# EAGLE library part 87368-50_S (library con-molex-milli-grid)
RECEPTACAL
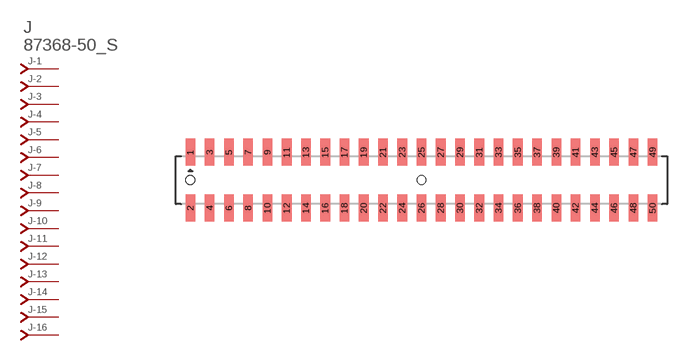
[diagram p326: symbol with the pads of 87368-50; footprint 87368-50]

Designator prefix J; gates -1=J-NV -2=J-N -3=J-N -4=J-N -5=J-N -6=J-N -7=J-N -8=J-N -9=J-N -10=J-N -11=J-N -12=J-N -13=J-N -14=J-N -15=J-N -16=J-N -17=J-N -18=J-N -19=J-N -20=J-N -21=J-N -22=J-N -23=J-N -24=J-N -25=J-N -26=J-N -27=J-N -28=J-N -29=J-N -30=J-N -31=J-N -32=J-N -33=J-N -34=J-N -35=J-N -36=J-N -37=J-N -38=J-N -39=J-N -40=J-N -41=J-N -42=J-N -43=J-N -44=J-N -45=J-N -46=J-N -47=J-N -48=J-N -49=J-N -50=J-N

## 87368-50_S  [87368-50]
1  -1:J  pas
2  -2:J  pas
3  -3:J  pas
4  -4:J  pas
5  -5:J  pas
6  -6:J  pas
7  -7:J  pas
8  -8:J  pas
9  -9:J  pas
10  -10:J  pas
11  -11:J  pas
12  -12:J  pas
13  -13:J  pas
14  -14:J  pas
15  -15:J  pas
16  -16:J  pas
17  -17:J  pas
18  -18:J  pas
19  -19:J  pas
20  -20:J  pas
21  -21:J  pas
22  -22:J  pas
23  -23:J  pas
24  -24:J  pas
25  -25:J  pas
26  -26:J  pas
27  -27:J  pas
28  -28:J  pas
29  -29:J  pas
30  -30:J  pas
31  -31:J  pas
32  -32:J  pas
33  -33:J  pas
34  -34:J  pas
35  -35:J  pas
36  -36:J  pas
37  -37:J  pas
38  -38:J  pas
39  -39:J  pas
40  -40:J  pas
41  -41:J  pas
42  -42:J  pas
43  -43:J  pas
44  -44:J  pas
45  -45:J  pas
46  -46:J  pas
47  -47:J  pas
48  -48:J  pas
49  -49:J  pas
50  -50:J  pas

## Footprint 87368-50 (pad centres in mm)
RECEPTACAL SMD Dual Row, Side Entry
smd 1 x 2.8: 1 -24,2.9; 2 -24,-2.9; 3 -22,2.9; 4 -22,-2.9; 5 -20,2.9; 6 -20,-2.9; 7 -18,2.9; 8 -18,-2.9; 9 -16,2.9; 10 -16,-2.9; 11 -14,2.9; 12 -14,-2.9; 13 -12,2.9; 14 -12,-2.9; 15 -10,2.9; 16 -10,-2.9; 17 -8,2.9; 18 -8,-2.9; 19 -6,2.9; 20 -6,-2.9; 21 -4,2.9; 22 -4,-2.9; 23 -2,2.9; 24 -2,-2.9; 25 0,2.9; 26 0,-2.9; 27 2,2.9; 28 2,-2.9; 29 4,2.9; 30 4,-2.9; 31 6,2.9; 32 6,-2.9; 33 8,2.9; 34 8,-2.9; 35 10,2.9; 36 10,-2.9; 37 12,2.9; 38 12,-2.9; 39 14,2.9; 40 14,-2.9; 41 16,2.9; 42 16,-2.9; 43 18,2.9; 44 18,-2.9; 45 20,2.9; 46 20,-2.9; 47 22,2.9; 48 22,-2.9; 49 24,2.9; 50 24,-2.9
hole 0.914 at -24,0
hole 0.914 at 0,0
